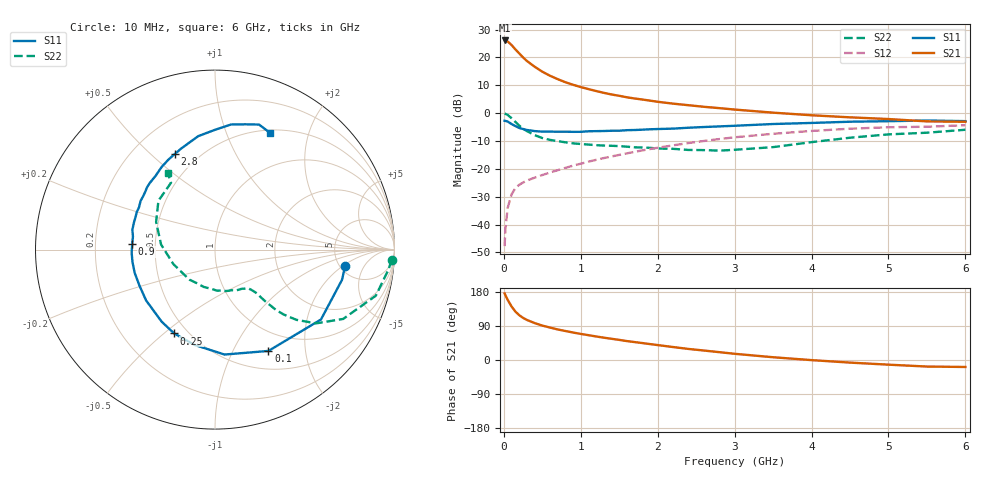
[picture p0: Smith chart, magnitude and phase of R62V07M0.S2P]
! SIEMENS Small Signal Semiconductors
! BFR193
! Si NPN RF Bipolar Junction Transistor in SOT23
! VCE = 2 V  IC = 7 mA
! Common Emitter S-Parameters:  May  1996
# GHz  S  MA  R  50
!  f  S11  S21  S12  S22
! GHz  MAG  ANG  MAG  ANG  MAG  ANG  MAG  ANG
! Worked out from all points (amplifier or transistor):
!   36 points, 10 MHz to 6 GHz, reference 50 ohm
!   highest |S21| = 26.1 dB at 10 MHz (marker M1)
!   |S21| within 3 dB of that: start of sweep to 143.5 MHz
!   unconditionally stable (mu >= 1): 800.4 MHz to 2 GHz
!   at 250 MHz: K = 0.53, MSG = 22.5 dB, |S12| = -24.9 dB
!   at 1.4 GHz: K = 1.05, MAG = 9.7 dB, |S12| = -15.6 dB
!   at 6 GHz: K = 0.96, MSG = 0.6 dB, |S12| = -4.3 dB
!   lowest NFmin = 1.20 dB at 450 MHz
!   S11 on the Smith chart (normalised r, x): 10 MHz: 5.60, -2.14; 100 MHz: 0.73, -1.39; 250 MHz: 0.42, -0.54; 900 MHz: 0.37, +0.03; 2.8 GHz: 0.37, +0.60; 6 GHz: 0.53, +1.44
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0.01  0.7313 -7.0  20.2 175.7  0.0041 87.1  0.9863 -3.3
0.02  0.7274 -13.4  19.86 171.2  0.0083 83.8  0.9728 -6.6
0.05  0.7073 -33.4  19.36 158.7  0.0199 75.1  0.9321 -16.0
0.1  0.6382 -62.2  16.74 141.4  0.0348 63.8  0.8121 -28.4
0.15  0.5872 -84.8  13.96 127.8  0.0452 56.5  0.6974 -36.1
0.2  0.543 -102.2  11.83 118.3  0.0518 53.1  0.5989 -40.8
0.25  0.5196 -116.0  10.02 111.1  0.0569 51.0  0.526 -43.4
0.3  0.4995 -126.5  8.645 105.7  0.0618 50.5  0.4771 -44.7
0.4  0.477 -143.6  6.826 97.5  0.0695 51.2  0.4036 -45.8
0.5  0.4663 -154.6  5.554 90.8  0.0776 53.2  0.3577 -46.2
0.6  0.466 -163.9  4.702 85.6  0.086 54.5  0.3318 -46.5
0.7  0.4649 -171.3  4.081 80.6  0.0948 55.8  0.315 -47.2
0.9  0.4624 176.1  3.235 72.5  0.1144 58.1  0.2874 -49.1
1.1  0.4734 166.6  2.706 65.5  0.1348 59.4  0.2731 -52.8
1.3  0.4783 158.0  2.316 58.9  0.1565 59.6  0.2624 -56.9
1.6  0.4954 146.8  1.927 49.9  0.1899 58.8  0.2502 -65.1
2.2  0.5281 128.7  1.483 34.2  0.2646 54.5  0.2291 -87.1
2.8  0.5786 112.6  1.232 20.7  0.343 47.2  0.2127 -118.9
3.5  0.6391 98.4  1.022 7.3  0.4268 36.6  0.2458 -160.9
4.5  0.7027 82.7  0.842 -6.9  0.5264 20.8  0.3626 154.8
5.5  0.7386 70.6  0.712 -17.3  0.5711 4.8  0.446 123.3
6  0.7196 64.9  0.701 -18.4  0.6076 0.0  0.5039 121.6
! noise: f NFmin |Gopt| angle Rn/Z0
0.45  1.2  0.24  125  0.12
0.9  1.25  0.36  154  0.11
1.8  2  0.55  -156  0.13
